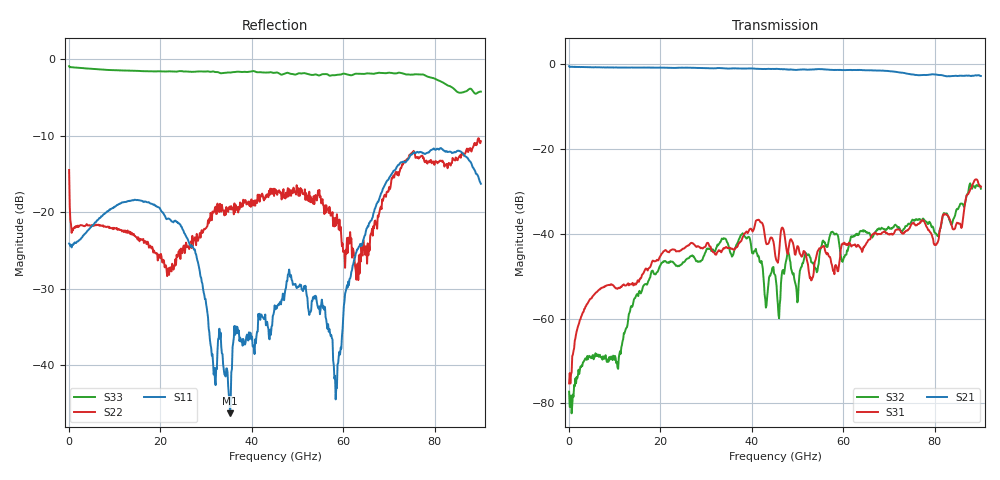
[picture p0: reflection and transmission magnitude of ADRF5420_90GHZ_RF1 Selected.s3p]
! Device:  ADRF5420
! Description: Flip-Chip, Silicon SPDT Switch
! Frequency:  0.1 GHz -  90 GHz
! Ports:
!  RFC = Port 1
!  RF1 = Port 2
!  RF2 = Port 3
! VDD  =  +3.3 Volts
! VSS  =  -3.3 Volts
! State
! RF1 Selected: CTRL = 3.3 V
! Data:  Data was collected using a calibrated network analyzer
!  The reference plane is the package boundry of ADRF5420 switch.
! Notes: Analog Devices supplies this data as a sample of measured data
!  for this product.  Your particular data for this product may vary.
!  Analog Devices reserves the right to change this data at anytime.
# GHz S  dB  R 50
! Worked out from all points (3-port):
!   656 points, 50 MHz to 90.07 GHz, reference 50 ohm
!   strongest paths, dB at 50 MHz, 22.59 GHz, 45.13 GHz, 67.67 GHz, 90.07 GHz:
!     S21: -0.5, -0.9, -1.1, -1.6, -2.8
!     S31: -75.3, -43.7, -45.2, -40.1, -28.9
!     S32: -77.2, -46.6, -49.8, -38.8, -29.4
!   lowest |S11| = -46.3 dB at 35.23 GHz (marker M1), VSWR 1.01, Z = 50.4 - j0.259 ohm
!   |S11| at or under -10 dB: start of sweep to end of sweep
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0.05  -24.10 -25.4  -0.65 1.0  -73.25 31.7
      -0.52 1.5  -14.47 43.3  -75.13 33.4
      -75.29 32.3  -77.23 -7.1  -0.90 -178.7
4.310562  -22.28 9.3  -0.74 -28.2  -55.90 61.6
          -0.77 -27.8  -21.72 -7.6  -69.32 26.2
          -55.99 61.5  -69.08 29.2  -1.22 156.4
15.443  -18.44 -36.2  -0.84 -99.9  -50.85 58.0
        -0.84 -97.7  -23.79 -54.2  -53.55 122.5
        -50.84 60.1  -53.47 122.2  -1.53 100.9
25.75081  -23.31 -100.8  -0.88 -167.4  -42.99 21.7
          -0.88 -163.8  -24.33 176.6  -45.98 28.5
          -42.96 24.7  -45.99 27.9  -1.60 52.9
35.234  -46.28 -32.0  -1.08 130.8  -43.28 -7.3
        -1.09 134.8  -19.24 83.9  -44.24 -62.5
        -43.31 -4.6  -44.31 -63.3  -1.74 12.1
45.1295  -32.69 -8.7  -1.15 65.1  -45.31 -86.3
         -1.15 70.6  -17.53 13.6  -49.86 -136.4
         -45.24 -81.7  -49.82 -138.3  -1.76 -31.3
58.46094  -42.92 117.3  -1.39 -25.8  -47.63 -129.9
          -1.41 -16.1  -20.95 -113.6  -40.07 85.4
          -47.60 -119.6  -39.98 84.3  -2.05 -88.6
68.49388  -17.25 -1.3  -1.67 -98.3  -39.73 167.6
          -1.56 -87.1  -18.32 -54.7  -38.73 11.4
          -39.73 177.0  -38.75 10.7  -1.77 -138.7
79.62631  -11.77 -100.3  -2.36 -178.8  -41.10 107.8
          -2.44 -167.1  -13.39 -99.1  -38.37 -61.7
          -41.26 117.3  -38.47 -62.5  -2.45 154.5
90.07156  -16.27 153.9  -3.32 98.1  -29.18 97.1
          -2.84 109.4  -10.72 -101.3  -29.21 -132.1
          -28.91 109.8  -29.40 -130.8  -4.23 85.8
